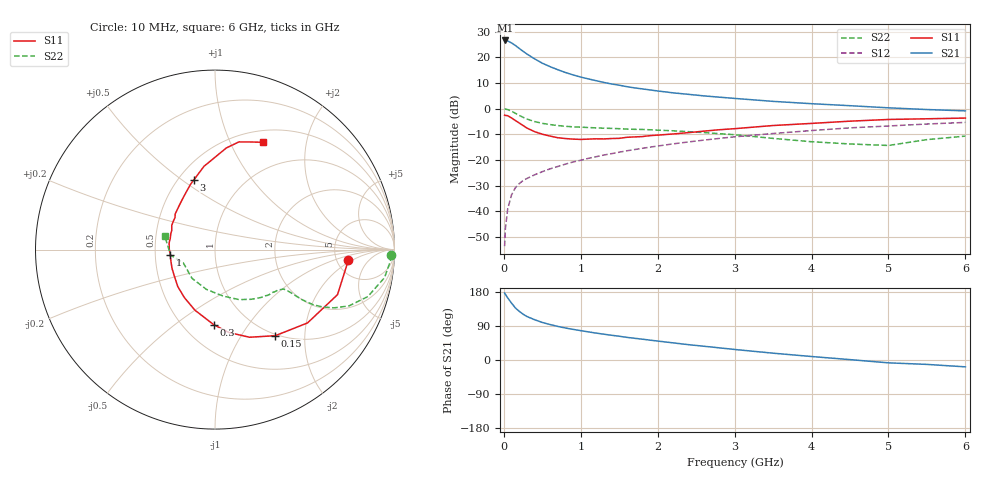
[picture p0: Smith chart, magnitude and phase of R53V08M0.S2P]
! SIEMENS Small Signal Semiconductors
! BFR183
! Si NPN RF Bipolar Junction Transistor in SOT23
! VCE = 3 V  IC = 8 mA
! Common Emitter S-Parameters:  May  1996
# GHz  S  MA  R  50
!  f  S11  S21  S12  S22
! GHz  MAG  ANG  MAG  ANG  MAG  ANG  MAG  ANG
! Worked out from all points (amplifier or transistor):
!   36 points, 10 MHz to 6 GHz, reference 50 ohm
!   highest |S21| = 26.5 dB at 20 MHz (marker M1)
!   |S21| within 3 dB of that: start of sweep to 195.6 MHz
!   unconditionally stable (mu >= 1): 849.6 MHz to 2.545 GHz
!   at 250 MHz: K = 0.55, MSG = 25.2 dB, |S12| = -28.0 dB
!   at 1.4 GHz: K = 1.06, MAG = 12.1 dB, |S12| = -17.5 dB
!   at 6 GHz: K = 0.89, MSG = 2.2 dB, |S12| = -5.4 dB
!   lowest NFmin = 1.30 dB at 450 MHz
!   S11 on the Smith chart (normalised r, x): 10 MHz: 6.45, -1.63; 150 MHz: 0.98, -1.43; 300 MHz: 0.69, -0.70; 1 GHz: 0.60, -0.04; 3 GHz: 0.60, +0.56; 6 GHz: 0.64, +1.33
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0.01  0.7458 -4.3  21.12 176.8  0.0021 82.7  0.9838 -1.9
0.02  0.736 -8.3  21.2 173.3  0.0046 83.2  0.9786 -3.9
0.05  0.7273 -20.2  20.73 164.0  0.0111 80.5  0.9573 -9.4
0.1  0.6577 -38.4  18.97 150.1  0.0209 73.6  0.8908 -17.1
0.15  0.5856 -55.0  16.92 137.4  0.0288 66.6  0.8097 -22.8
0.2  0.5248 -68.5  14.84 128.5  0.0346 63.5  0.7378 -26.1
0.25  0.4684 -80.5  13.03 120.9  0.0398 61.5  0.6776 -28.1
0.3  0.4181 -91.0  11.56 114.8  0.0436 60.9  0.6277 -29.3
0.4  0.3557 -108.3  9.291 106.3  0.0514 60.6  0.5593 -29.9
0.5  0.3173 -122.5  7.655 99.1  0.0592 61.0  0.5164 -29.8
0.6  0.2921 -135.3  6.558 93.6  0.0671 61.6  0.4887 -29.6
0.7  0.2711 -146.3  5.724 88.7  0.0746 62.5  0.4681 -29.6
0.8  0.2615 -156.1  5.048 84.5  0.083 62.7  0.453 -29.7
1  0.2512 -173.7  4.109 77.4  0.0988 63.2  0.4351 -30.5
1.1  0.2548 179.5  3.781 74.2  0.1077 63.4  0.4282 -31.4
1.6  0.2764 150.6  2.675 59.7  0.151 62.0  0.3994 -36.7
2.2  0.3207 127.4  2.027 45.2  0.2057 57.8  0.3699 -46.1
3  0.4068 106.7  1.579 27.8  0.2822 49.9  0.3102 -64.1
3.5  0.4683 97.5  1.383 18.0  0.3273 43.8  0.2631 -80.0
4.5  0.5693 83.7  1.139 1.0  0.4218 31.7  0.2049 -128.7
5.5  0.6337 71.1  0.959 -11.6  0.5011 19.6  0.249 -172.7
6  0.6542 66.0  0.903 -18.1  0.5383 11.7  0.2915 164.4
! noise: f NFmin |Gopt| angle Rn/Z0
0.45  1.3  0.17  43  0.21
0.9  1.35  0.21  115  0.2
1.8  2.05  0.33  -177  0.14
